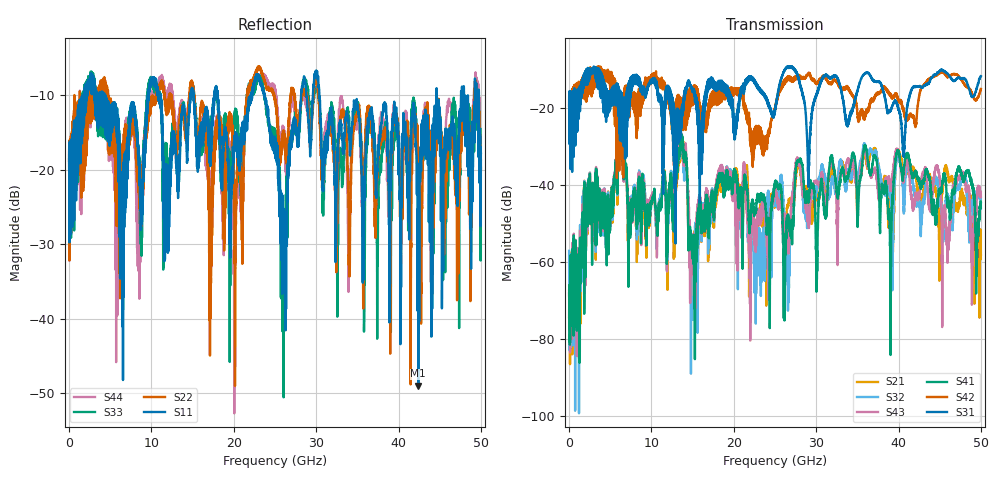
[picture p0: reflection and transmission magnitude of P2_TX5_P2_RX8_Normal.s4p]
!Keysight Technologies,N5225B,MY57041031,A.13.20.10
!Date: Friday, May 31, 2019 11:39:38
!Correction: S11(Full 4 Port(1,2,3,4))
!S12(Full 4 Port(1,2,3,4))
!S13(Full 4 Port(1,2,3,4))
!S14(Full 4 Port(1,2,3,4))
!S21(Full 4 Port(1,2,3,4))
!S22(Full 4 Port(1,2,3,4))
!S23(Full 4 Port(1,2,3,4))
!S24(Full 4 Port(1,2,3,4))
!S31(Full 4 Port(1,2,3,4))
!S32(Full 4 Port(1,2,3,4))
!S33(Full 4 Port(1,2,3,4))
!S34(Full 4 Port(1,2,3,4))
!S41(Full 4 Port(1,2,3,4))
!S42(Full 4 Port(1,2,3,4))
!S43(Full 4 Port(1,2,3,4))
!S44(Full 4 Port(1,2,3,4))
!S4P File: Measurements: <S11,S12,S13,S14>,
!<S21,S22,S23,S24>,
!<S31,S32,S33,S34>,
!<S41,S42,S43,S44>:
# Hz S  dB  R 50.0
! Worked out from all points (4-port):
!   5000 points, 10 MHz to 50 GHz, reference 50 ohm
!   strongest paths, dB at 10 MHz, 12.51 GHz, 25.01 GHz, 37.51 GHz, 50 GHz:
!     S31: -19.4, -17.8, -21.0, -13.2, -11.8
!     S42: -19.5, -21.6, -20.1, -16.3, -15.1
!     S41: -68.3, -45.8, -39.1, -37.2, -44.5
!     S43: -67.6, -45.9, -40.5, -41.7, -43.2
!     S32: -57.2, -43.1, -44.6, -34.5, -46.0
!     S21: -74.5, -44.1, -44.5, -34.5, -58.2
!   lowest |S11| = -49.0 dB at 42.4 GHz (marker M1), VSWR 1.01, Z = 49.7 + j0.101 ohm
!   |S11| at or under -10 dB: 4.421 GHz to 9.569 GHz (5.148 GHz wide, 73.6 % of centre); 23.73 GHz to 28.18 GHz (4.441 GHz wide, 17.1 % of centre); 30.39 GHz to 44.61 GHz (14.22 GHz wide, 37.9 % of centre)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
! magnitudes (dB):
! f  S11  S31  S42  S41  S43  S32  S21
! 10 MHz  -19.8  -19.4  -19.5  -68.3  -67.6  -57.2  -74.5
! 6.29 GHz  -29.2  -24.2  -27.9  -28.7  -28.5  -28.7  -29.0
! 13.65 GHz  -12.9  -20.4  -18.6  -27.0  -26.7  -27.2  -27.6
! 14.94 GHz  -9.6  -15.3  -14.6  -57.5  -59.0  -68.6  -59.8
! 18.46 GHz  -18.4  -13.1  -16.5  -37.2  -34.9  -36.0  -37.9
! 42.4 GHz  -49.0  -14.4  -18.5  -38.6  -43.3  -44.0  -42.4
! 50 GHz  -19.9  -11.8  -15.1  -44.5  -43.2  -46.0  -58.2
